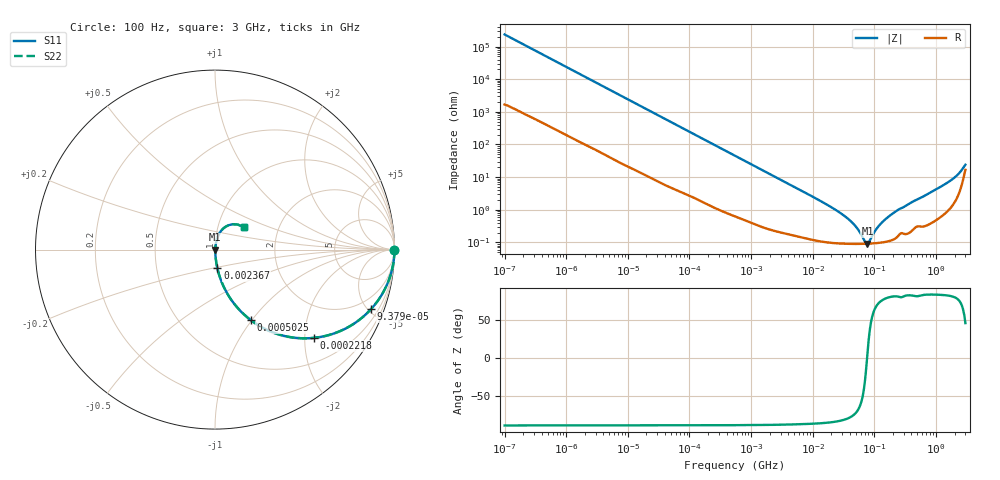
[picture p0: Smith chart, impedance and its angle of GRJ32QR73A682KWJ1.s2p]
!Murata Part Number: GRJ32QR73A682KWJ1
!These Parameters are Measured in Series Mode Connection
!Data Generated on Jun 19, 2026
!  o--ll--o
!Port1  Port2
!  o------o
!Operation Temp=25[degC], DC Bias Voltage=0[V]
!Freq. Start=100[Hz] Stop=3[GHz] 401[Steps]
# Hz S RI R 50
!Freq.(Hz) S11(Real) S11(Imag) S21(Real) S21(Imag) S12(Real) S12(Imag) S22(Real) S22(Imag)
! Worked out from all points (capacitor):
!   401 points, 100 Hz to 3 GHz, reference 50 ohm
!   read as one part in series: C = 6.75 nF near 109 Hz
!   lowest |Z| = 91.4 mohm at 77.31 MHz (marker M1)
!   series resonance near 76.21 MHz, so ESL is about 650 pH
!   S11 on the Smith chart (normalised r, x): 100 Hz: open; 93.79 kHz: 1.06, -5.21; 221.8 kHz: 1.03, -2.22; 502.5 kHz: 1.01, -0.98; 2.367 MHz: 1.00, -0.21; 3 GHz: 1.33, +0.34
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100  1 -0.000425  3.2e-06 0.000425  3.2e-06 0.000425  1 -0.000425
1788  0.9999 -0.00748  0.000118 0.00748  0.000118 0.00748  0.9999 -0.00748
10443  0.9978 -0.0431  0.00224 0.0431  0.00224 0.0431  0.9978 -0.0431
31977  0.9818 -0.1291  0.0182 0.1291  0.0182 0.1291  0.9818 -0.1291
93790  0.869 -0.332  0.131 0.332  0.131 0.332  0.869 -0.332
221826  0.551 -0.4916  0.449 0.4916  0.449 0.4916  0.551 -0.4916
502545  0.1983 -0.392  0.8017 0.392  0.8017 0.392  0.1983 -0.392
547723  0.173 -0.3714  0.827 0.3714  0.827 0.3714  0.173 -0.3714
1000599  0.0615 -0.2324  0.9385 0.2324  0.9385 0.2324  0.0615 -0.2324
2366551  0.0132 -0.1041  0.9868 0.1041  0.9868 0.1041  0.0132 -0.1041
9794414  0.00184 -0.0255  0.9982 0.0255  0.9982 0.0255  0.00184 -0.0255
2.21892e7  0.00106 -0.0105  0.9989 0.0105  0.9989 0.0105  0.00106 -0.0105
3.71925e7  0.000927 -0.00524  0.9991 0.00524  0.9991 0.00524  0.000927 -0.00524
5.248048e7  0.0009 -0.00256  0.9991 0.00256  0.9991 0.00256  0.0009 -0.00256
7.093284e7  0.000903 -0.000481  0.9991 0.000481  0.9991 0.000481  0.000903 -0.000481
7.730952e7  0.000908 9.77e-05  0.9991 -9.77e-05  0.9991 -9.77e-05  0.000908 9.77e-05
1.188943e8  0.000972 0.0031  0.999 -0.0031  0.999 -0.0031  0.000972 0.0031
1.751444e8  0.00114 0.0063  0.9989 -0.0063  0.9989 -0.0063  0.00114 0.0063
2.471375e8  0.00172 0.00998  0.9983 -0.00998  0.9983 -0.00998  0.00172 0.00998
1.506733e9  0.0127 0.0643  0.9873 -0.0643  0.9873 -0.0643  0.0127 0.0643
2.317205e9  0.0417 0.1134  0.9583 -0.1134  0.9583 -0.1134  0.0417 0.1134
3e9  0.1614 0.1235  0.8386 -0.1235  0.8386 -0.1235  0.1614 0.1235
